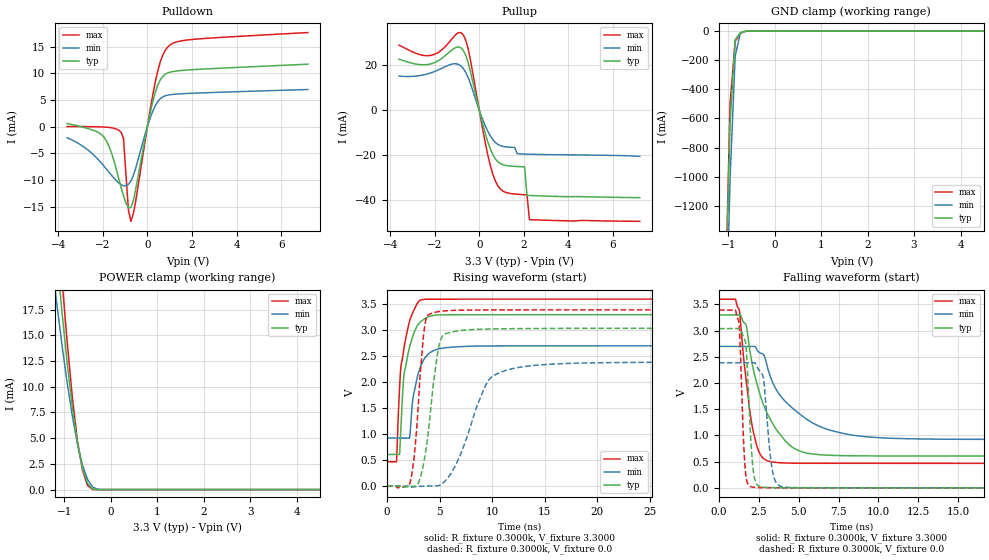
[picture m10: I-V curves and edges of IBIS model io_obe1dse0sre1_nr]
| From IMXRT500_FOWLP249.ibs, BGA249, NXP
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[Model] io_obe1dse0sre1_nr
|   Model io_obe1dse0sre1_nr
| Library cells for typ/min/max conditions are connected as defined below:
|  pad - External Pad
|  ipp_do - Core Input
|  ipp_obe - Output Buffer Enable
|  REFH3V3 - vdd1v8
|  REFL3V3 - REFL3V3
|  gnde - gnde
|  ipp_ina235_3v - NC
|  ipp_ina40_3v - NC
|  ipp_ina_mux - NC
|  ipp_ind - NC
|  ipp_ind_1p8v - NC
|  ipp_ind_3v - NC
|  ipp_sre - vdd
|  vdd - vdd
|  vdd1v8 - vdd1v8
|  vdda - vdde3v3
|  vdde3v3 - vdde3v3
| All other pins connected to ground
Model_type I/O
Polarity   Non-Inverting
Enable   Active-High
Vinl =   0.9900V
Vinh =   2.3100V
Vmeas =  1.6500V
Cref =   25.0000pF
Rref =   0.5000k
Vref =   0.0V
C_comp   1.8910pF   1.8218pF   2.0891pF
[Temperature Range]   25.0000   0.1250k   -40.0000
[Voltage Range]   3.3000V   2.7000V   3.6000V
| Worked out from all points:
|   slope of the pulldown table from 0 to 0.495 V, typ, clamps not added: 61.4 ohm
|   slope of the pullup table from 0 to 0.495 V, typ, clamps not added: 28.7 ohm
|   GND clamp passes 1 mA (typ) near -0.55 V on its own axis
|   POWER clamp passes 1 mA (typ) near -0.53 V on its own axis
|   rising waveform, R_fixture 0.3000k, V_fixture 3.3000: 20-80 % time 945ps typ, 994ps min, 889ps max; typ from 0.608 V to 3.3 V
|   rising waveform, R_fixture 0.3000k, V_fixture 0.0: 20-80 % time 1.08ns typ, 2.6ns min, 748ps max; typ from 0 V to 3.04 V
|   falling waveform, R_fixture 0.3000k, V_fixture 3.3000: 20-80 % time 1.66ns typ, 2.65ns min, 742ps max; typ from 3.3 V to 0.608 V
|   falling waveform, R_fixture 0.3000k, V_fixture 0.0: 20-80 % time 313ps typ, 419ps min, 248ps max; typ from 3.04 V to 0 V
[Pulldown]
|Voltage   I(typ)   I(min)   I(max)
-3.6V     580uA      -2.07mA    30uA
-1.95V    -1.94mA    -7.35mA    -60uA
-1.62V    -4.76mA    -9.02mA    -180uA
-1.18V    -11.35mA   -10.84mA   -1.013mA
-1.07V    -12.94mA   -11.04mA   -2.193mA
-850mV    -15.13mA   -10.79mA   -15.56mA
-740mV    -15.14mA   -10.18mA   -17.69mA
-520mV    -11.65mA   -7.709mA   -13.83mA
360mV     6.495mA    3.971mA    8.469mA
580mV     8.787mA    5.251mA    12.13mA
910mV     10.06mA    5.911mA    14.9mA
7.2V      11.7mA     6.966mA    17.62mA
[Pullup]
|Voltage   I(typ)   I(min)   I(max)
-3.6V     22.77mA    15.22mA    29.02mA
-2.15V    20.76mA    16.76mA    24.51mA
-1.05V    28mA       20.75mA    33.76mA
-720mV    26.73mA    18.68mA    33.68mA
-500mV    21.29mA    14.62mA    27.43mA
160mV     -6.397mA   -4.301mA   -8.846mA
600mV     -19.59mA   -12.99mA   -28.27mA
1.04V     -24.21mA   -16.05mA   -35.92mA
2.03V     -25.25mA   -19.52mA   -37.65mA
2.14V     -37.93mA   -19.55mA   -37.71mA
2.25V     -37.98mA   -19.58mA   -48.76mA
7.2V      -38.97mA   -20.58mA   -49.5mA
[GND_clamp]
|Voltage   I(typ)   I(min)   I(max)
-3.6V     -46.64A    -46.27A    -48.09A
-1.07V    -2.038A    -2.424A    -1.965A
-960mV    -629.9mA   -1.012A    -499.2mA
-850mV    -61.62mA   -174.1mA   -72.03mA
-740mV    -13.6mA    -15.68mA   -16.3mA
-630mV    -2.659mA   -3.244mA   -3.911mA
-410mV    -9.214uA   -49.17uA   -3.123uA
7.2V      0A         0A         0A
[POWER_clamp]
|Voltage   I(typ)   I(min)   I(max)
-3.6V     124.7mA    103.4mA    137.3mA
-1.27V    28.14mA    22.17mA    33.67mA
-1.16V    22.5mA     17.97mA    26.85mA
-1.05V    17.19mA    14.01mA    20.36mA
-940mV    12.34mA    10.39mA    14.37mA
-830mV    8.067mA    7.189mA    9.044mA
-720mV    4.554mA    4.475mA    4.783mA
-610mV    2.051mA    2.374mA    1.895mA
-500mV    596.8uA    974uA      390.7uA
-390mV    63.25uA    246uA      14.24uA
-170mV    55.4nA     1.772uA    16.57nA
7.2V      0A         0A         0A
[Ramp]
| variable   typ   min   max
dV/dt_r  0.7575/1.5657n   0.5823/5.4982n   1.1236/1.2689n
dV/dt_f  0.3253/1.8692n   0.1897/2.4816n   0.4971/1.0882n
R_load = 50.0000
[Rising Waveform]
R_fixture= 0.3000k
V_fixture= 3.3000
V_fixture_min= 2.7000
V_fixture_max= 3.6000
|time   V(typ)   V(min)   V(max)
0s        607.6mV    923.7mV    467.4mV
903.4ps   607.6mV    923.7mV    472.6mV
1.192ns   615.1mV    923.7mV    1.886V
1.324ns   1.175V     923.7mV    2.303V
1.595ns   2.1V       923.7mV    2.633V
2.137ns   2.669V     921.5mV    3.168V
2.52ns    2.923V     1.749V     3.371V
3.614ns   3.224V     2.468V     3.596V
11.04ns   3.3V       2.699V     3.6V
500ns     3.3V       2.7V       3.6V
[Rising Waveform]
R_fixture= 0.3000k
V_fixture= 0.0
V_fixture_min= 0.0
V_fixture_max= 0.0
|time   V(typ)   V(min)   V(max)
0s        91.73nV    1.941uV    241.1nV
2.141ns   -11.02mV   -4.771mV   34.46mV
2.56ns    -7.058mV   -17.07mV   519.9mV
2.998ns   65.38mV    -8.387mV   1.63V
3.763ns   780.5mV    -2.629mV   3.246V
4.978ns   2.727V     9.772mV    3.363V
6.399ns   2.977V     350.7mV    3.384V
9.991ns   3.026V     2.109V     3.392V
19.31ns   3.037V     2.371V     3.394V
500ns     3.038V     2.386V     3.394V
[Falling Waveform]
R_fixture= 0.3000k
V_fixture= 3.3000
V_fixture_min= 2.7000
V_fixture_max= 3.6000
|time   V(typ)   V(min)   V(max)
0s        3.3V       2.7V       3.6V
1.27ns    3.299V     2.7V       3.399V
1.71ns    3.101V     2.7V       2.048V
1.922ns   2.658V     2.7V       1.499V
2.492ns   1.869V     2.592V     701.6mV
3.327ns   1.25V      2.041V     494.8mV
4.462ns   808.6mV    1.562V     471.9mV
7.941ns   613.5mV    1.03V      467.4mV
15.37ns   607.7mV    926.3mV    467.4mV
500ns     607.6mV    923.7mV    467.4mV
[Falling Waveform]
R_fixture= 0.3000k
V_fixture= 0.0
V_fixture_min= 0.0
V_fixture_max= 0.0
|time   V(typ)   V(min)   V(max)
0s        3.038V     2.386V     3.394V
1.25ns    3.038V     2.386V     3.162V
1.655ns   2.802V     2.386V     330.3mV
2.136ns   378.9mV    2.386V     12.11mV
2.641ns   19.04mV    2.198V     3.628mV
2.796ns   12.36mV    2.082V     2.741mV
3.173ns   6.031mV    747.3mV    1.45mV
3.449ns   4.199mV    202.6mV    934.2uV
4.951ns   998uV      5.169mV    103uV
500ns     1.151uV    3.186uV    894.9nV
